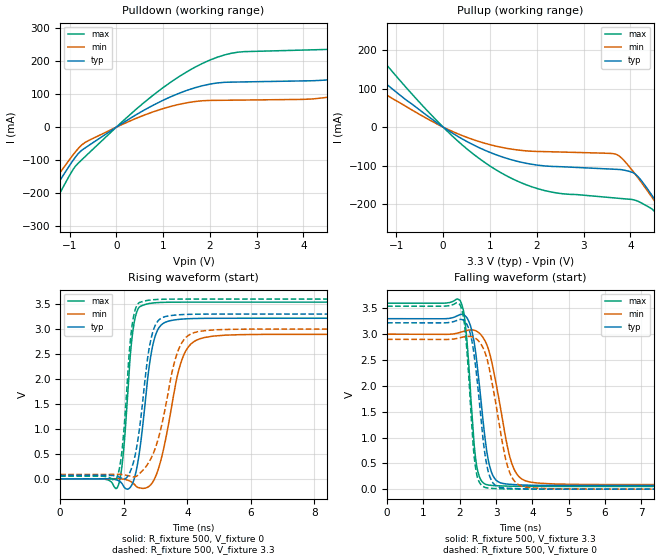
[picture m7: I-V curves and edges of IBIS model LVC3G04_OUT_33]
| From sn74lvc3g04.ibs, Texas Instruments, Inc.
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[Model]   LVC3G04_OUT_33
Model_type  Output
Vref =   0
Rref =   500
Cref =   50p
Vmeas =   1.5
| variable   typ   min   max
C_comp   9.49pF   5.86pF   12.60pF
| C_pullup   9.85pF   5.86pF   11.98pF
| C_pulldown   9.13pF   6.35pF   12.60pF
[Temperature Range]   40   100   -40
| Ambient temperature   25   85   -40
[Voltage range]   3.3   3   3.6
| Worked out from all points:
|   slope of the pulldown table from 0 to 0.495 V, typ, clamps not added: 11.3 ohm
|   slope of the pullup table from 0 to 0.495 V, typ, clamps not added: 13.6 ohm
|   rising waveform, R_fixture 500, V_fixture 0: 20-80 % time 365ps typ, 548ps min, 248ps max; typ from 0 V to 3.22 V
|   falling waveform, R_fixture 500, V_fixture 3.3: 20-80 % time 311ps typ, 467ps min, 215ps max; typ from 3.3 V to 0.069 V
|   rising waveform, R_fixture 500, V_fixture 3.3: 20-80 % time 382ps typ, 610ps min, 252ps max; typ from 0.069 V to 3.3 V
|   falling waveform, R_fixture 500, V_fixture 0: 20-80 % time 302ps typ, 447ps min, 207ps max; typ from 3.22 V to 0 V
[Pulldown]
| LVC3G04_OUT_33
|   Voltage   I(typ)   I(min)   I(max)
-5V       -1.007A    -894.5mA   -1.188A
-2.44V    -443.8mA   -389mA     -531.5mA
-1.495V   -228mA     -197.1mA   -278.2mA
-570mV    -53.91mA   -39.16mA   -76.55mA
975mV     79.99mA    55.23mA    117.5mA
2.315V    136.3mA    81.67mA    219.5mA
4.95V     154.8mA    103mA      243.8mA
6.98V     278.7mA    201.5mA    397.1mA
7.35V     308.5mA    129.4mA    437.7mA
7.84V     330.1mA    92.49mA    494.9mA
8.635V    176.4mA    93.08mA    532.7mA
10V       158.4mA    95.01mA    294.8mA
[Pullup]
| LVC3G04_OUT_33
|   Voltage   I(typ)   I(min)   I(max)
-5V       547.6mA    429.5mA    769.3mA
-3.23V    334.2mA    258.6mA    474.2mA
-2.495V   249.6mA    191.6mA    356.4mA
-1.985V   193mA      147.1mA    277.1mA
-95mV     7.957mA    5.812mA    11.78mA
1.095V    -70.05mA   -48.34mA   -108.1mA
2.165V    -100.6mA   -63.48mA   -164.5mA
3.71V     -109.5mA   -71.26mA   -184.2mA
4.145V    -126.1mA   -128.6mA   -191.4mA
4.775V    -234.9mA   -237.1mA   -267.2mA
5.015V    -281mA     -280.3mA   -317.6mA
10V       -1.311A    -1.23A     -1.479A
[Ramp]
| LVC3G04_OUT_33
| variable   typ   min   max
dV/dt_r   2.05/3.96E-10   1.85/5.91E-10   2.24/2.70E-10
dV/dt_f   1.99/3.24E-10   1.80/4.87E-10   2.18/2.28E-10
R_load = 500
[Rising Waveform]
| LVC3G04_OUT_33
R_fixture =   500
C_fixture =   0
L_fixture =   0
V_fixture =   0
V_fixture_min = 0
V_fixture_max = 0
|   Time   V(typ)   V(min)   V(max)
0s        141.8pV    5.06nV     2.398nV
1.81ns    -29.64mV   3.124mV    -159.7mV
1.975ns   -124.1mV   -4.506mV   432.8mV
2.32ns    -20.15mV   -101.6mV   3.096V
2.745ns   1.965V     -170.6mV   3.503V
2.94ns    2.745V     -35.28mV   3.523V
3.175ns   3.079V     388.4mV    3.533V
3.83ns    3.199V     2.385V     3.538V
4.535ns   3.214V     2.829V     3.539V
24.99ns   3.216V     2.894V     3.539V
[Falling Waveform]
| LVC3G04_OUT_33
R_fixture =   500
C_fixture =   0
L_fixture =   0
V_fixture =   3.3
V_fixture_min = 3
V_fixture_max = 3.6
|   Time   V(typ)   V(min)   V(max)
0s        3.3V       3V         3.6V
2.015ns   3.381V     3.036V     3.647V
2.175ns   3.338V     3.067V     3.057V
2.325ns   3.091V     3.083V     1.582V
2.46ns    2.53V      3.059V     483.5mV
2.79ns    551.2mV    2.708V     79.75mV
3ns       174.4mV    2.048V     67.39mV
3.415ns   92.31mV    539.1mV    57.7mV
3.98ns    75.68mV    133mV      54.26mV
24.99ns   69.39mV    87.32mV    53.21mV
[Rising Waveform]
| LVC3G04_OUT_33
R_fixture =   500
C_fixture =   0
L_fixture =   0
V_fixture =   3.3
V_fixture_min = 3
V_fixture_max = 3.6
|   Time   V(typ)   V(min)   V(max)
0s        69.35mV    87.26mV    53.17mV
1.775ns   51.41mV    89.98mV    9.118mV
1.96ns    7.058mV    84.47mV    656.7mV
2.285ns   286.8mV    40.03mV    3.165V
2.67ns    1.988V     219.7mV    3.563V
2.86ns    2.806V     411.7mV    3.583V
3.08ns    3.164V     789.9mV    3.593V
3.7ns     3.283V     2.549V     3.599V
4.335ns   3.297V     2.948V     3.6V
24.99ns   3.3V       3V         3.6V
[Falling Waveform]
| LVC3G04_OUT_33
R_fixture =   500
C_fixture =   0
L_fixture =   0
V_fixture =   0
V_fixture_min = 0
V_fixture_max = 0
|   Time   V(typ)   V(min)   V(max)
0s        3.22V      2.9V       3.542V
2.015ns   3.286V     2.932V     3.56V
2.16ns    3.232V     2.952V     3.001V
2.305ns   2.978V     2.955V     1.527V
2.43ns    2.414V     2.922V     447.9mV
2.725ns   545.7mV    2.585V     28.89mV
2.915ns   119.6mV    1.966V     13.58mV
3.32ns    18.77mV    434.7mV    4.55mV
3.82ns    5.918mV    38.94mV    1.259mV
24.99ns   36.3uV     46.09uV    29.99uV
